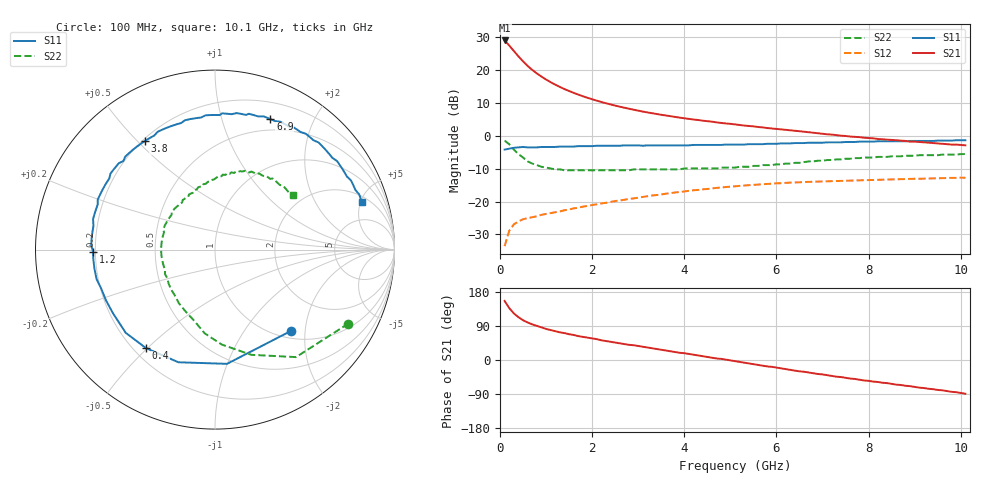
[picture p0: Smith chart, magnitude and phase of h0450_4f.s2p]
!HBFP-0450
!S and NOISE PARAMETERS at Vce=4V  Ic=20mA.  LAST UPDATED  09-04-98
# GHZ S MA R  50
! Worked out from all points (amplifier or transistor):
!   101 points, 100 MHz to 10.1 GHz, reference 50 ohm
!   highest |S21| = 29.1 dB at 100 MHz (marker M1)
!   |S21| within 3 dB of that: start of sweep to 288 MHz
!   unconditionally stable (mu >= 1): 2.425 GHz to end of sweep
!   at 1.7 GHz: K = 0.87, MSG = 17.2 dB, |S12| = -21.8 dB
!   at 5.1 GHz: K = 1.10, MAG = 7.5 dB, |S12| = -15.3 dB
!   at 10.1 GHz: K = 1.04, MAG = 3.6 dB, |S12| = -12.7 dB
!   lowest NFmin = 1.35 dB at 1.8 GHz
!   S11 on the Smith chart (normalised r, x): 100 MHz: 1.14, -1.68; 400 MHz: 0.25, -0.50; 1.2 GHz: 0.19, -0.01; 3.8 GHz: 0.21, +0.52; 6.9 GHz: 0.37, +1.44; 10.1 GHz: 2.51, +5.12
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0.1  0.62 -47.0  28.45 156.0  0.021 62.0  0.85 -29.0
0.2  0.64 -84.0  23.86 137.0  0.036 51.0  0.75 -53.0
0.3  0.66 -108.0  19.68 123.0  0.045 44.0  0.62 -71.0
0.4  0.67 -125.0  16.28 113.0  0.05 38.0  0.53 -86.0
0.5  0.68 -137.0  13.69 105.0  0.054 35.0  0.47 -97.0
0.6  0.67 -148.0  11.63 99.0  0.056 33.0  0.41 -107.0
0.7  0.67 -155.0  10.13 94.0  0.058 32.0  0.38 -116.0
0.8  0.67 -161.0  8.95 90.0  0.06 32.0  0.36 -124.0
0.9  0.68 -166.0  8.01 86.0  0.063 31.0  0.34 -131.0
1  0.68 -171.0  7.23 82.0  0.065 31.0  0.33 -138.0
1.2  0.68 -179.0  6.04 76.0  0.069 31.0  0.31 -149.0
1.5  0.69 172.0  4.83 68.0  0.076 31.0  0.3 -162.0
1.8  0.7 164.0  4.02 61.0  0.084 30.0  0.3 -173.0
2.2  0.71 155.0  3.29 52.0  0.094 29.0  0.3 175.0
2.5  0.71 148.0  2.9 46.0  0.102 27.0  0.3 168.0
3.5  0.72 129.0  2.1 27.0  0.129 19.0  0.31 148.0
3.8  0.72 123.0  1.95 21.0  0.138 17.0  0.31 143.0
5.1  0.74 100.0  1.5 -3.0  0.171 1.0  0.33 117.0
6.8  0.79 69.0  1.12 -35.0  0.201 -22.0  0.41 85.0
6.9  0.79 67.0  1.1 -37.0  0.202 -24.0  0.42 84.0
8.5  0.83 42.0  0.87 -63.0  0.218 -44.0  0.49 60.0
10.1  0.86 18.0  0.72 -89.0  0.231 -67.0  0.53 35.0
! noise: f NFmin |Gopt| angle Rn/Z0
1.8  1.35  0.47  -165  0.06
2  1.4  0.49  -163  0.06
2.5  1.53  0.52  -151  0.09
3.5  1.79  0.58  -132  0.19
4  1.91  0.63  -121  0.29
5  2.17  0.68  -102  0.56
5.5  2.3  0.7  -92  0.8
7  2.68  0.76  -64  1.78
8  2.94  0.8  -47  2.73
10  3.44  0.83  -18  4.69
